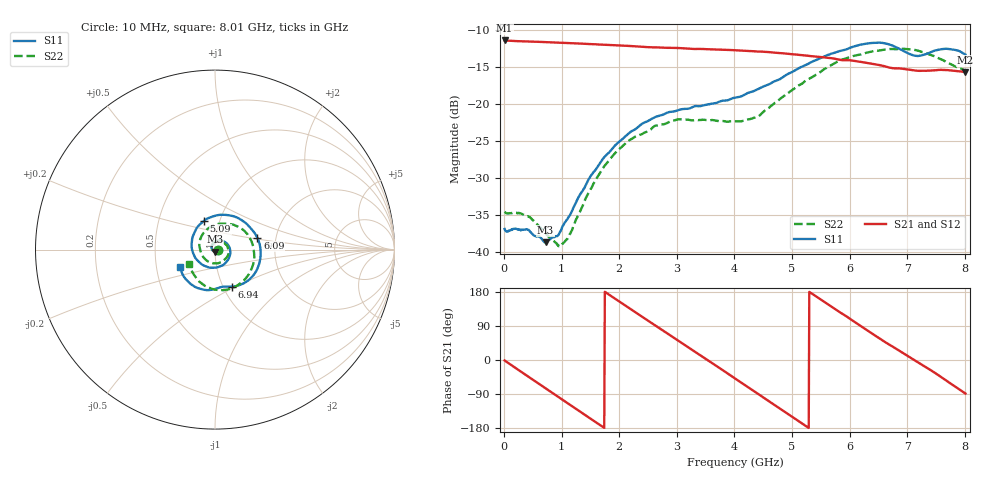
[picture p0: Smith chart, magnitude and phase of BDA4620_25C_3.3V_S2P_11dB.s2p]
!Agilent Technologies,E5071B,MY42404982,A.09.10
!Date: Wed May 06 08:50:47 2026
!Data & Calibration Information:
!Freq	S11:SOLT2(ON)	S21:SOLT2(ON)	S12:SOLT2(ON)	S22:SOLT2(ON)
# Hz S RI R 50
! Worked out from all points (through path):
!   801 points, 10 MHz to 8.01 GHz, reference 50 ohm
!   highest |S21| = -11.43 dB at 10 MHz (marker M1); lowest = -15.7 dB at 8.01 GHz (marker M2)
!   group delay of S21, straight-line fit = 280 ps
!   lowest |S11| = -38.7 dB at 720 MHz (marker M3), VSWR 1.02, Z = 49.9 - j1.16 ohm
!   |S11| at or under -10 dB: start of sweep to end of sweep
!   |S22| runs from -39.2 to -12.5 dB; largest |S21 - S12| = 0.0012
!   S11 on the Smith chart (normalised r, x): 10 MHz: 1.03, -0.00; 5.09 GHz: 0.84, +0.28; 6.09 GHz: 1.60, +0.22; 6.94 GHz: 1.10, -0.48; 8.01 GHz: 0.67, -0.13
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1e7  0.0144 -0.00096  0.268 -0.0058  0.2684 -0.00582  0.0188 -0.00112
4.3e8  0.01 -0.01  0.1869 -0.1862  0.1871 -0.1866  0.0137 -0.0108
7.2e8  -0.00099 -0.0116  0.0685 -0.2522  0.0685 -0.2527  0.00309 -0.0133
9.9e8  -0.0132 -0.00504  -0.0561 -0.2526  -0.0564 -0.2531  -0.00867 -0.00707
1.35e9  -0.0194 0.0167  -0.1938 -0.1659  -0.194 -0.1662  -0.0155 0.0126
1.64e9  -0.00876 0.0376  -0.2473 -0.0483  -0.2475 -0.0483  -0.0082 0.032
1.94e9  0.0159 0.0508  -0.2346 0.0826  -0.2349 0.0828  0.0126 0.0456
2.33e9  0.0568 0.041  -0.1256 0.2093  -0.1259 0.2097  0.0472 0.0394
2.68e9  0.083 0.00522  0.017 0.24  0.0174 0.2403  0.0704 0.0141
3.39e9  0.0396 -0.0884  0.2276 0.0585  0.228 0.0582  0.0462 -0.0628
4.01e9  -0.0736 -0.0822  0.1521 -0.1729  0.1522 -0.1734  -0.0451 -0.062
4.52e9  -0.1304 0.02  -0.0418 -0.221  -0.0421 -0.2214  -0.0873 0.0208
5.09e9  -0.0616 0.1603  -0.2007 -0.0771  -0.2011 -0.0771  -0.0185 0.1301
5.35e9  0.0162 0.1921  -0.209 0.0193  -0.2092 0.0195  0.0464 0.1443
5.68e9  0.1305 0.1749  -0.1589 0.1275  -0.1589 0.1278  0.1334 0.1247
6.09e9  0.2364 0.0646  -0.0339 0.1921  -0.034 0.1924  0.2101 0.0268
6.39e9  0.2504 -0.0618  0.0643 0.1752  0.0645 0.1754  0.2166 -0.0651
6.68e9  0.1853 -0.1718  0.1326 0.1163  0.1331 0.1165  0.1792 -0.1506
6.94e9  0.0956 -0.206  0.1649 0.0501  0.1654 0.0501  0.1153 -0.2054
7.19e9  0.0378 -0.2072  0.1663 -0.0189  0.1669 -0.0187  0.0321 -0.2269
7.58e9  -0.0771 -0.2202  0.1219 -0.1182  0.1223 -0.1185  -0.0807 -0.1841
8.01e9  -0.1929 -0.096  0.0046 -0.1636  0.00462 -0.1639  -0.1458 -0.0819
